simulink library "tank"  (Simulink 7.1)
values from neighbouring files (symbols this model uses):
  g = 981    [define_process.m]    (also in dyntester.m)
  k = 1.6    [define_process.m]    (also in dyntester.m = mean(k))
  kc = 10/16    (= 0.625)    [define_process.m]    (also in dyntester.m = 0.588235294118)
libraries: tank x4

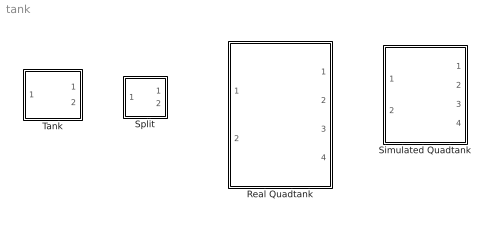
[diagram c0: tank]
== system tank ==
  Real Quadtank : Subsystem  AncestorBlock=tank/Real Quadtank  mask{h=0.05}
  Simulated Quadtank : Subsystem  mask{gamma1=0.7, gamma2=0.7}
  Split : Subsystem  mask{g=}
      mask prompts: g "gamma"
  Tank : Subsystem  mask{h0=10, a=0.03, A1=4.9, g=981}
      mask prompts: h0 "h0 [cm]"; a "a [cm^2]"; A1 "A [cm^ 2]"; g "g [cm/s^2]"

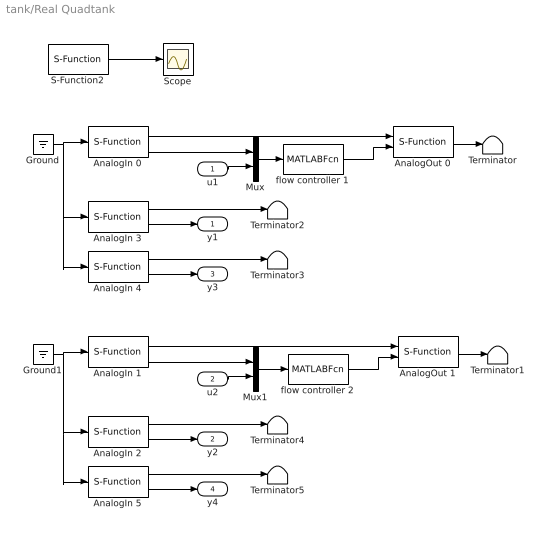
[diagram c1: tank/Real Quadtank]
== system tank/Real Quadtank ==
  u1 : Inport  OutDataType=sfix(16)  OutScaling=2^0
  u2 : Inport  Port=2  OutDataType=sfix(16)  OutScaling=2^0
  AnalogIn 0 : S-Function  FunctionName=analogin  Parameters=h [35]  EnableBusSupport=off
  AnalogIn 1 : S-Function  FunctionName=analogin  Parameters=h [34]  EnableBusSupport=off
  AnalogIn 2 : S-Function  FunctionName=analogin  Parameters=h [33]  EnableBusSupport=off
  AnalogIn 3 : S-Function  FunctionName=analogin  Parameters=h [31]  EnableBusSupport=off
  AnalogIn 4 : S-Function  FunctionName=analogin  Parameters=h [30]  EnableBusSupport=off
  AnalogIn 5 : S-Function  FunctionName=analogin  Parameters=h [32]  EnableBusSupport=off
  AnalogOut 0 : S-Function  FunctionName=analogout  Parameters=h [31]  EnableBusSupport=off
  AnalogOut 1 : S-Function  FunctionName=analogout  Parameters=h [30]  EnableBusSupport=off
  Ground : Ground
  Ground1 : Ground
  Mux : Mux  Inputs=2
  Mux1 : Mux  Inputs=2
  S-Function2 : S-Function  FunctionName=realtimer  Parameters=h  EnableBusSupport=off
  Scope : Scope
  Terminator{,1..5} (6 alike) : Terminator
  flow controller 1 : MATLABFcn  MATLABFcn=flowCtrl1  SampleTime=0.01
  flow controller 2 : MATLABFcn  MATLABFcn=flowCtrl2  SampleTime=0.01
  y1 : Outport  OutDataType=sfix(16)  OutScaling=2^0
  y2 : Outport  Port=2  OutDataType=sfix(16)  OutScaling=2^0
  y3 : Outport  Port=3  OutDataType=sfix(16)  OutScaling=2^0
  y4 : Outport  Port=4  OutDataType=sfix(16)  OutScaling=2^0
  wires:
  AnalogIn 0/2 -> Mux/1
  AnalogIn 1/2 -> Mux1/1
  flow controller 2/1 -> AnalogOut 1/2
  Mux1/1 -> flow controller 2/1
  u2/1 -> Mux1/2
  flow controller 1/1 -> AnalogOut 0/2
  Mux/1 -> flow controller 1/1
  u1/1 -> Mux/2
  AnalogIn 5/1 -> Terminator5/1
  AnalogIn 2/1 -> Terminator4/1
  Ground1/1 -> AnalogIn 1/1, AnalogIn 2/1, AnalogIn 5/1
  AnalogIn 5/2 -> y4/1
  AnalogIn 2/2 -> y2/1
  AnalogIn 4/1 -> Terminator3/1
  AnalogIn 3/1 -> Terminator2/1
  Ground/1 -> AnalogIn 4/1, AnalogIn 3/1, AnalogIn 0/1
  AnalogIn 4/2 -> y3/1
  AnalogIn 3/2 -> y1/1
  AnalogOut 1/1 -> Terminator1/1
  AnalogIn 1/1 -> AnalogOut 1/1
  AnalogOut 0/1 -> Terminator/1
  AnalogIn 0/1 -> AnalogOut 0/1
  S-Function2/1 -> Scope/1

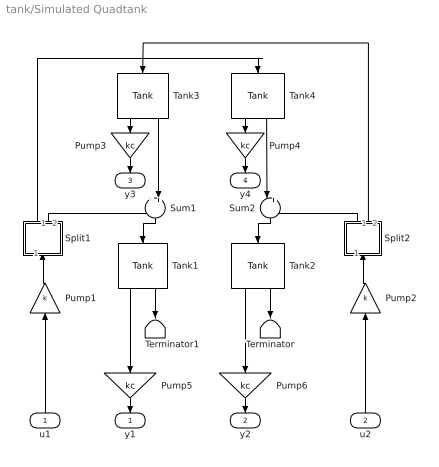
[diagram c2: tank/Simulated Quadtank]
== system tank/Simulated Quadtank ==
  u1 : Inport  Orientation=up
  u2 : Inport  Orientation=up  Port=2
  Pump1 : Gain  Orientation=up  Gain=k
  Pump2 : Gain  Orientation=up  Gain=k
  Pump{3..6} (4 alike) : Gain  Orientation=down  Gain=kc
  Split1 : Subsystem  Orientation=up  AncestorBlock=tank/Split  mask{g1=gamma1}
      mask prompts: g1 "gamma1"
  Split2 : Subsystem  Orientation=up  AncestorBlock=tank/Split  mask{g2=gamma2}
      mask prompts: g2 "gamma2"
  Sum1 : Sum  Orientation=down  Inputs=++|
  Sum2 : Sum  Orientation=down  Inputs=|++
  Tank{1..4} (4 alike) : tank/Tank  Orientation=down  SystemSampleTime=-1  h0=0  a=a  A1=A  g=g
  Terminator : Terminator
  Terminator1 : Terminator
  y1 : Outport  Orientation=down
  y2 : Outport  Orientation=down  Port=2
  y3 : Outport  Orientation=down  Port=3
  y4 : Outport  Orientation=down  Port=4
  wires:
  Split2/2(1-g2) -> Tank3/1
  Tank4/2 -> Sum2/1
  Sum2/1 -> Tank2/1
  Pump2/1 -> Split2/1(" ")
  Split2/1(g2) -> Sum2/2
  Split1/1(1-g1) -> Tank4/1
  Tank2/2 -> Terminator/1
  Tank1/2 -> Terminator1/1
  Sum1/1 -> Tank1/1
  Tank3/2 -> Sum1/2
  Pump1/1 -> Split1/1(" ")
  u1/1 -> Pump1/1
  u2/1 -> Pump2/1
  Split1/2(g1) -> Sum1/1
  Tank3/1 -> Pump3/1
  Pump3/1 -> y3/1
  Tank4/1 -> Pump4/1
  Pump4/1 -> y4/1
  Tank1/1 -> Pump5/1
  Tank2/1 -> Pump6/1
  Pump5/1 -> y1/1
  Pump6/1 -> y2/1

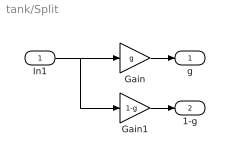
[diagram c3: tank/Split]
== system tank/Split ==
  In1 : Inport
  Gain : Gain  Gain=g
  Gain1 : Gain  Gain=1-g
  g : Outport
  1-g : Outport  Port=2
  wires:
  Gain1/1 -> 1-g/1
  Gain/1 -> g/1
  In1/1 -> Gain1/1, Gain/1

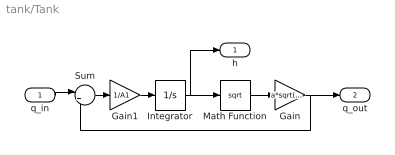
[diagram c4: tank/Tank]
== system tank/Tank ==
  q_in : Inport
  Gain : Gain  Gain=a*sqrt(2*g)
  Gain1 : Gain  Gain=1/A1
  Integrator : Integrator  InitialCondition=h0  LimitOutput=on  UpperSaturationLimit=16  LowerSaturationLimit=0
  Math Function : Math  Operator=sqrt  OutputSignalType=real
  Sum : Sum  Inputs=|+-
  h : Outport
  q_out : Outport  Port=2
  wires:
  q_in/1 -> Sum/1
  Integrator/1 -> Math Function/1, h/1
  Math Function/1 -> Gain/1
  Gain/1 -> q_out/1, Sum/2
  Sum/1 -> Gain1/1
  Gain1/1 -> Integrator/1

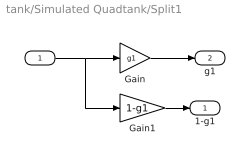
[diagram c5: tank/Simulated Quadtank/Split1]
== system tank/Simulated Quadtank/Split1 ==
  " " : Inport
  Gain : Gain  Gain=g1
  Gain1 : Gain  Gain=1-g1
  1-g1 : Outport
  g1 : Outport  Port=2
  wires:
  " "/1 -> Gain/1, Gain1/1
  Gain1/1 -> 1-g1/1
  Gain/1 -> g1/1

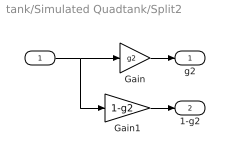
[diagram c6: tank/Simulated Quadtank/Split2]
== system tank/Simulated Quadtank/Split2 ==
  " " : Inport
  Gain : Gain  Gain=g2
  Gain1 : Gain  Gain=1-g2
  g2 : Outport
  1-g2 : Outport  Port=2
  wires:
  " "/1 -> Gain/1, Gain1/1
  Gain/1 -> g2/1
  Gain1/1 -> 1-g2/1
